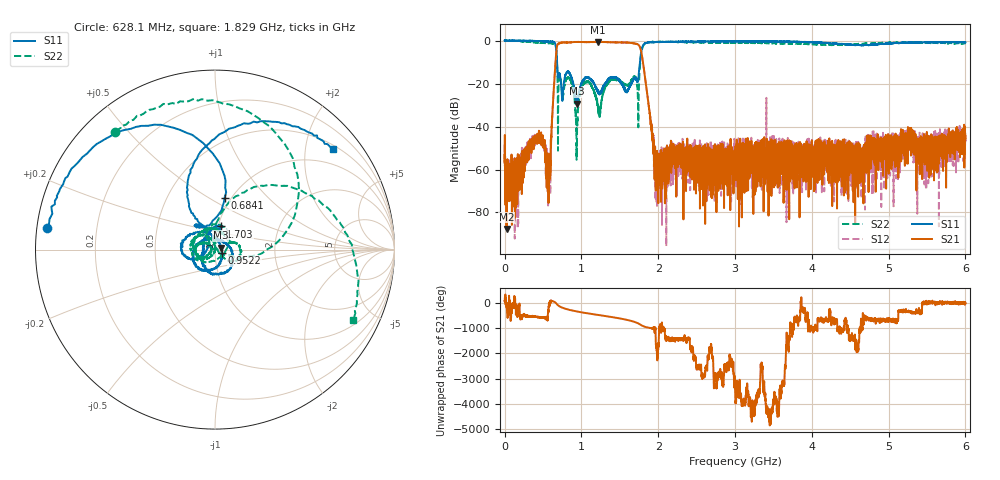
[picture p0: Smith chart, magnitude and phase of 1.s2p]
#  HZ  S  MA  R  50.00
! Rohde & Schwarz Vector Network Analyzer
! Rohde-Schwarz,ZNL6-2Port,1323001206101378,1.50.1.34-21.10.1.104
! Created: UTC 3/8/2024, 2:25:20 AM
! freq[Hz]  mag:S11  ang:S11  mag:S21  ang:S21  mag:S12  ang:S12  mag:S22  ang:S22
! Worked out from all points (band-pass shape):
!   6000 points, 5 kHz to 6 GHz, reference 50 ohm
!   highest |S21| = -0.57 dB at 1.216 GHz (marker M1); lowest = -87.6 dB at 25.01 MHz (marker M2)
!   |S21| within 3 dB of the highest: 678.1 MHz to 1.768 GHz (1.09 GHz wide, 89.1 % of centre)
!   lowest |S11| = -29.4 dB at 941.2 MHz (marker M3), VSWR 1.07, Z = 53.3 + j1.24 ohm
!   |S11| at or under -10 dB: 683.4 MHz to 1.761 GHz (1.078 GHz wide, 88.2 % of centre)
!   |S22| runs from -55.4 to 0.1 dB; largest |S21 - S12| = 0.048
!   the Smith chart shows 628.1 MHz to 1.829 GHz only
!   S11 on the Smith chart (normalised r, x): 628.1 MHz: 0.03, +0.06; 684.1 MHz: 0.93, +0.59; 952.2 MHz: 1.08, -0.04; 1.703 GHz: 1.03, +0.27; 1.829 GHz: 0.58, +2.60
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5000  1.007 -0.5  0.00219 63.4  0.003817 60.2  1.006 -0.5
2.500915e7  0.998 -5.5  4.157e-05 -83.3  0.0003335 -136.1  1.002 -6.9
3.200581e8  0.9988 -73.4  0.002502 -159.1  0.003413 -164.0  0.9349 -91.3
5.690994e8  0.9553 -154.8  0.0005903 67.6  0.001265 -30.3  0.8699 176.5
6.281092e8  0.9413 172.6  0.03012 53.8  0.02968 54.6  0.86 130.2
6.841184e8  0.2946 79.5  0.7677 -69.4  0.7642 -69.4  0.2623 -4.5
7.501294e8  0.04559 154.8  0.9056 163.7  0.8997 161.6  0.05945 -5.9
8.281423e8  0.1939 169.8  0.9067 87.4  0.906 86.7  0.1344 167.1
9.411611e8  0.03395 20.0  0.9302 12.6  0.9327 10.9  0.001893 -84.1
9.521629e8  0.0421 -24.5  0.934 6.4  0.9347 4.4  0.01978 -112.2
1.000171e9  0.1035 -88.5  0.9273 -19.4  0.9308 -22.0  0.08189 -138.1
1.216207e9  0.0606 108.1  0.9361 -123.5  0.934 -124.3  0.02902 139.1
1.360231e9  0.1323 -47.1  0.9176 169.1  0.9141 168.7  0.1096 -173.4
1.510255e9  0.113 -124.9  0.9079 92.6  0.9034 91.9  0.1104 90.1
1.703287e9  0.1326 76.6  0.8504 -50.0  0.848 -50.6  0.1387 -20.5
1.768298e9  0.4117 111.6  0.6628 -144.0  0.656 -144.5  0.3477 65.1
1.829308e9  0.8644 40.5  0.1344 124.9  0.1365 125.1  0.8646 -27.0
2.000337e9  0.9232 -27.6  0.001824 11.2  0.001226 -57.5  0.9364 -117.9
3.000503e9  0.961 -101.7  0.001178 -114.8  0.002365 63.5  0.8997 98.3
4.000668e9  0.9187 -119.7  0.00333 8.8  0.002229 45.5  0.8298 27.8
5.000834e9  0.8626 -119.0  0.0008554 9.0  0.004006 9.9  0.8872 -29.8
6e9  0.9193 -131.7  0.005974 -46.0  0.006097 -2.6  0.8759 -88.8
